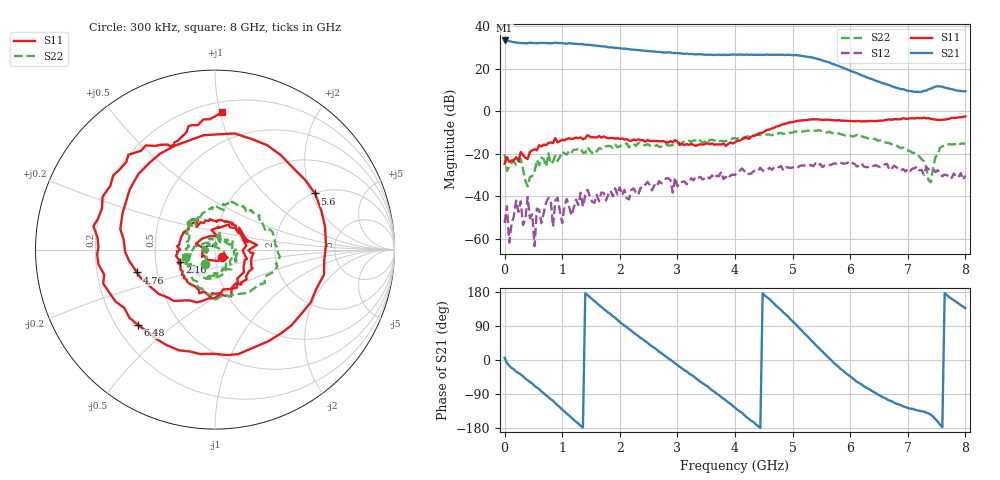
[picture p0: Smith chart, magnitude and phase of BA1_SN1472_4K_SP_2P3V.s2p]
! VC=2.3V IC=16.36mA
# HZ S DB R 50.00
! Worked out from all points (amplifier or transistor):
!   201 points, 300 kHz to 8 GHz, reference 50 ohm
!   highest |S21| = 33.4 dB at 300 kHz (marker M1)
!   |S21| within 3 dB of that: start of sweep to 1.768 GHz
!   unconditionally stable (mu >= 1): start of sweep to 2.96 GHz; 2.96 GHz to 3.595 GHz; 6.219 GHz to end of sweep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
!   at 1.32 GHz: K = 1.19, MAG = 32.3 dB, |S12| = -38.3 dB
!   at 4 GHz: K = 0.96, MSG = 28.3 dB, |S12| = -29.9 dB
!   at 8 GHz: K = 2.12, MAG = 13.8 dB, |S12| = -30.2 dB
!   S11 on the Smith chart (normalised r, x): 300 kHz: 1.08, -0.09; 2.16 GHz: 0.67, -0.10; 4.76 GHz: 0.38, -0.12; 5.6 GHz: 2.01, +2.13; 6.48 GHz: 0.29, -0.38; 8 GHz: 0.27, +1.01
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300000  -24.64 -47.3  33.42 5.9  -52.54 12.2  -20.10 -124.9
8.0297e7  -23.85 -78.5  33.15 -15.1  -61.75 -121.0  -26.20 -159.6
2.002925e8  -21.61 -150.6  32.46 -30.8  -41.98 -59.4  -25.17 -154.9
6.40276e8  -16.51 56.2  32.29 -82.9  -52.58 113.4  -21.73 80.0
8.80267e8  -12.56 6.3  32.39 -114.1  -42.02 120.8  -20.86 36.3
1.120258e9  -12.63 -26.3  32.15 -146.6  -45.20 28.1  -18.63 -0.3
1.360249e9  -13.14 -58.1  31.65 -178.2  -44.89 -35.3  -19.47 -20.5
1.720236e9  -11.75 -109.9  30.61 134.5  -38.43 30.0  -16.65 -83.5
2.160219e9  -13.71 -160.2  29.32 82.0  -41.41 2.6  -16.90 -144.5
2.6802e9  -14.07 152.8  28.06 22.0  -32.82 -58.5  -16.67 174.0
2.960189e9  -13.48 128.0  27.57 -8.5  -31.12 -107.3  -15.22 149.2
3.400172e9  -15.45 78.1  26.90 -57.8  -30.83 -144.5  -13.91 131.9
4.00015e9  -14.58 -31.6  26.75 -126.0  -29.94 -174.0  -12.55 94.2
4.440134e9  -10.15 -109.3  26.72 -179.2  -26.51 140.9  -11.17 61.8
4.760122e9  -6.88 -163.7  26.65 137.0  -26.25 109.2  -10.27 37.2
5.08011e9  -4.45 135.5  26.49 90.5  -26.66 74.5  -9.47 13.1
5.360099e9  -3.66 80.4  25.28 46.8  -25.82 45.9  -8.95 -11.2
5.60009e9  -3.89 29.3  23.37 9.4  -25.22 32.3  -10.01 -29.0
5.920078e9  -4.45 -37.3  20.10 -34.1  -24.53 -1.2  -11.36 -66.9
6.480057e9  -4.43 -135.5  14.13 -90.7  -25.85 -63.9  -13.81 -119.2
6.68005e9  -3.73 -163.2  12.41 -107.1  -27.51 -89.0  -14.90 -142.8
8e9  -2.32 87.1  9.49 136.7  -30.20 -173.6  -15.30 -165.3
